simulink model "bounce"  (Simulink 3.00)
settings: Solver=ode23  SolverMode=SingleTasking  StartTime=0.0  StopTime=20  MaxStep=.01  RelTol=1e-3  AbsTol=1e-6

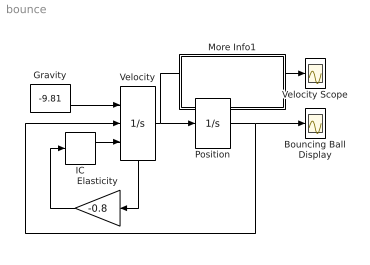
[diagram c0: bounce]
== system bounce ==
  Bouncing Ball Display : Scope
  Elasticity : Gain  Orientation=left  Gain=-0.8  SaturateOnIntegerOverflow=on
  Gravity : Constant  Value=-9.81
  IC : InitialCondition  Value=15
  More Info1 : Subsystem
  Position : Integrator  ExternalReset=none  InitialConditionSource=internal  InitialCondition=10  LimitOutput=on  UpperSaturationLimit=inf  LowerSaturationLimit=0  ShowSaturationPort=off  ShowStatePort=off  AbsoluteTolerance=auto
  Velocity : Integrator  ExternalReset=falling  InitialConditionSource=external  InitialCondition=0  LimitOutput=off  UpperSaturationLimit=inf  LowerSaturationLimit=-inf  ShowSaturationPort=off  ShowStatePort=on  AbsoluteTolerance=auto
  Velocity Scope : Scope
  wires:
  Velocity/State -> Elasticity/1
  IC/1 -> Velocity/3
  Elasticity/1 -> IC/1
  Velocity/1 -> Position/1, Velocity Scope/1
  Position/1 -> Bouncing Ball Display/1, Velocity/2
  Gravity/1 -> Velocity/1

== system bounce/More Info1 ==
